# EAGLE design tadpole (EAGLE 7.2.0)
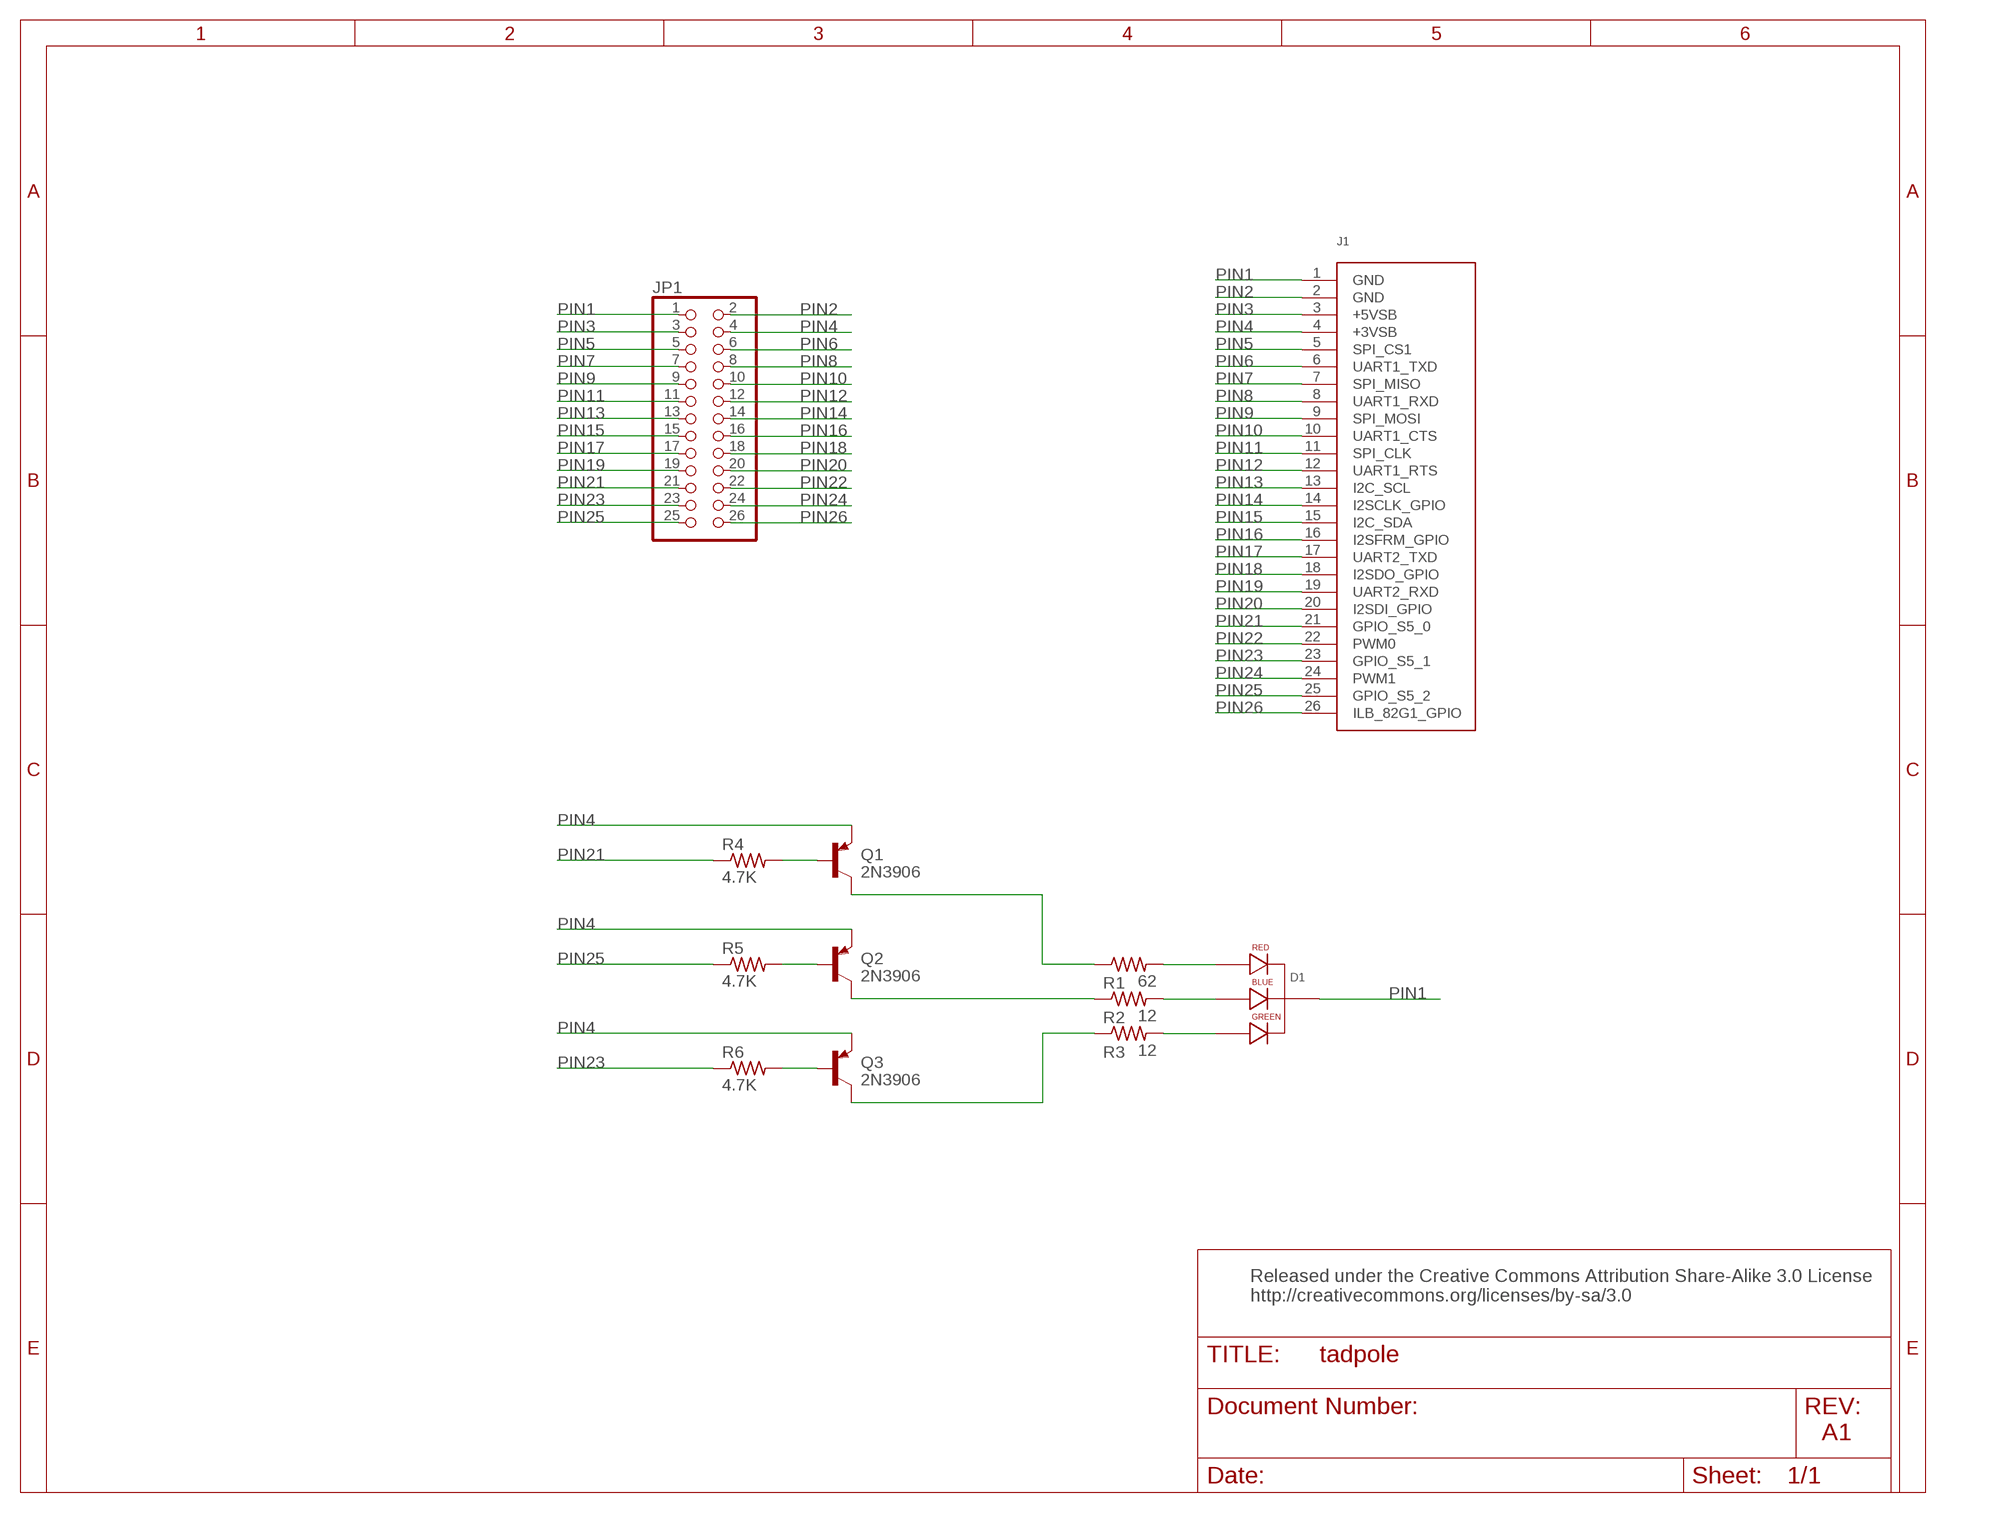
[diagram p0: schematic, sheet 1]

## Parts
D1  LED-RGB-CC-THRUCLEAR  [LED-RGB-THRU]
J1  MBM_LSE  [MBM_LSE]
JP1  PINHD-2X13  [2X13]
Q1  2N3906  [TO92]
Q2  2N3906  [TO92]
Q3  2N3906  [TO92]
R1  62  R-US_0204/5  [0204/5]
R2  12  R-US_0204/5  [0204/5]
R3  12  R-US_0204/5  [0204/5]
R4  4.7K  R-US_0204/5  [0204/5]
R5  4.7K  R-US_0204/5  [0204/5]
R6  4.7K  R-US_0204/5  [0204/5]

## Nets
N$1: Q1.1(C) R1.1
N$2: Q2.1(C) R2.1
N$3: Q3.1(C) R3.1
N$4: Q1.2(B) R4.2
N$5: Q2.2(B) R5.2
N$6: Q3.2(B) R6.2
N$105: D1.1(RED_CATHODE) R1.2
N$106: D1.3(GREEN_CATHODE) R2.2
N$107: D1.4(BLUE_CATHODE) R3.2
PIN1: D1.2(CATHODE) J1.1(GND) JP1.1
PIN2: J1.2(GND) JP1.2
PIN3: J1.3(+5VSB) JP1.3
PIN4: J1.4(+3VSB) JP1.4 Q1.3(E) Q2.3(E) Q3.3(E)
PIN5: J1.5(SPI_CS1) JP1.5
PIN6: J1.6(UART1_TXD) JP1.6
PIN7: J1.7(SPI_MISO) JP1.7
PIN8: J1.8(UART1_RXD) JP1.8
PIN9: J1.9(SPI_MOSI) JP1.9
PIN10: J1.10(UART1_CTS) JP1.10
PIN11: J1.11(SPI_CLK) JP1.11
PIN12: J1.12(UART1_RTS) JP1.12
PIN13: J1.13(I2C_SCL) JP1.13
PIN14: J1.14(I2SCLK_GPIO) JP1.14
PIN15: J1.15(I2C_SDA) JP1.15
PIN16: J1.16(I2SFRM_GPIO) JP1.16
PIN17: J1.17(UART2_TXD) JP1.17
PIN18: J1.18(I2SDO_GPIO) JP1.18
PIN19: J1.19(UART2_RXD) JP1.19
PIN20: J1.20(I2SDI_GPIO) JP1.20
PIN21: J1.21(GPIO_S5_0) JP1.21 R4.1
PIN22: J1.22(PWM0) JP1.22
PIN23: J1.23(GPIO_S5_1) JP1.23 R6.1
PIN24: J1.24(PWM1) JP1.24
PIN25: J1.25(GPIO_S5_2) JP1.25 R5.1
PIN26: J1.26(ILB_82G1_GPIO) JP1.26

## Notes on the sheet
- Released under the Creative Commons Attribution Share-Alike 3.0 License
  http://creativecommons.org/licenses/by-sa/3.0
- A1

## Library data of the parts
D1 = SparkFun-LED:LED-RGB-CC-THRU: RGB Through-hole common cathode LED SparkFun Storefront: COM-00105 (Clear) COM-09264 (Diffuse); PROD_ID: DIO-08418
J1 = mini-lse-lure:MBM_LSE
JP1 = pinhead:PINHD-2X13: PIN HEADER
Q1-Q3 = transistor-pnp:2N3906: PNP Transistor
R1-R6 = resistor:R-US_: RESISTOR, American symbol

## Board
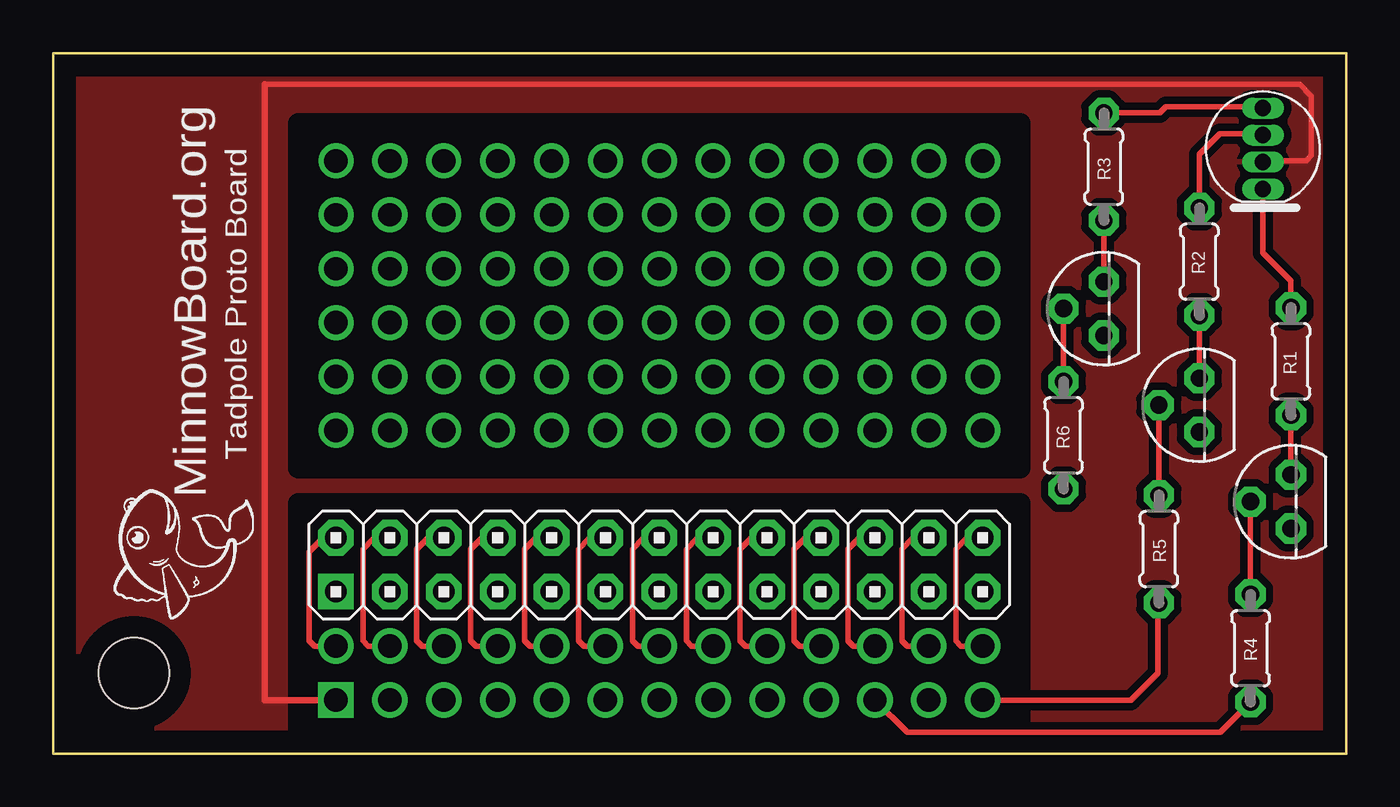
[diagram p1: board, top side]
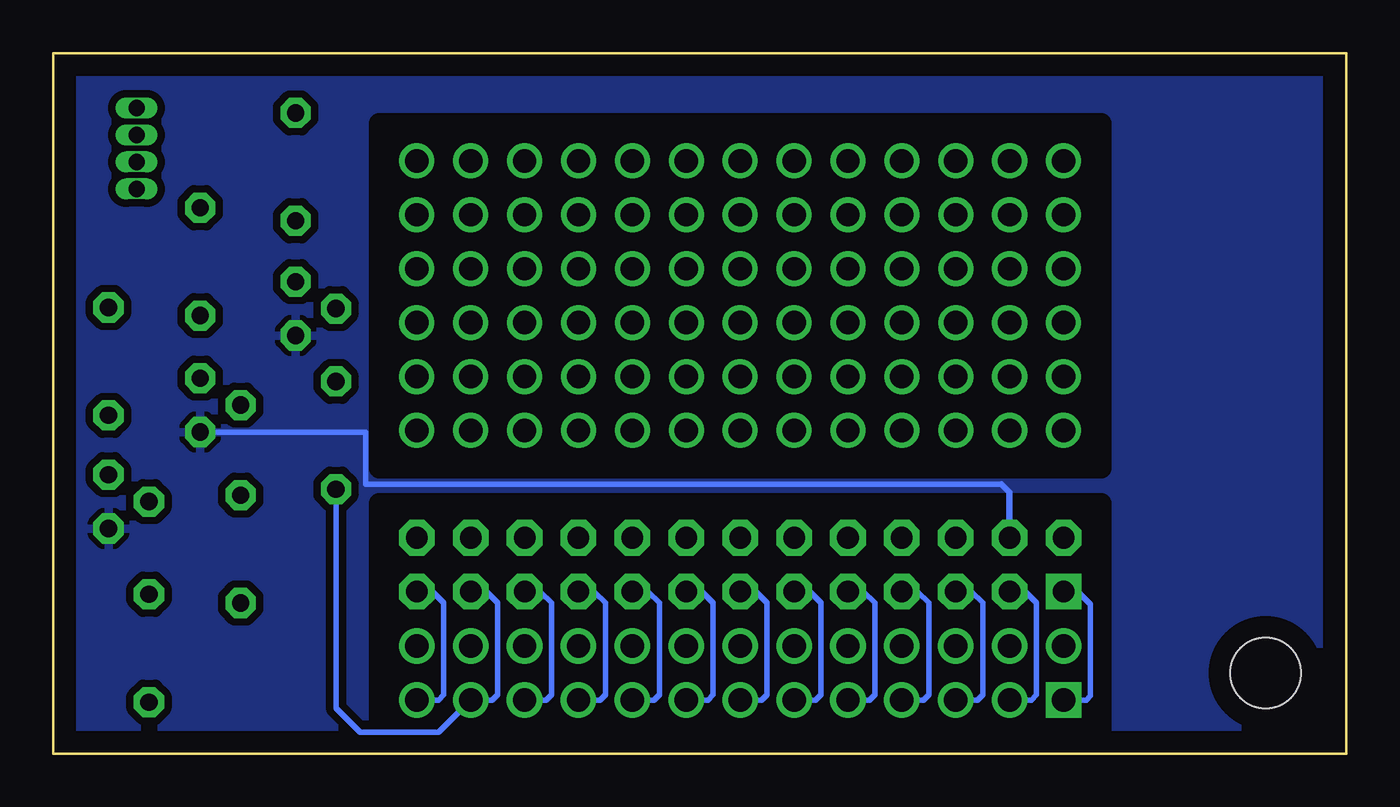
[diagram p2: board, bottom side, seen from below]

Size 60.96 x 33.02 mm. Coordinates in mm from the lower left corner, seen from the top.
Copper layers (1*16): Top 0.035mm / dielectric 1.5mm / Bottom 0.035mm
Design rules "default *": minimum track width 10mil, minimum drill 24mil, track to track 10mil, track to pad 10mil, pad to pad 10mil, via to via 10mil, smd to smd 8mil, copper to edge 40mil, drill to drill 8mil, minimum pad ring 0mil, minimum via ring 8mil, stop-mask expansion 4mil, vias tented up to drill 0mil, thermal gap 10mil
tRestrict: area 11.6,13.5 to 45.6,29.7; area 11.6,0.2 to 45.6,11.8
bRestrict: area 11.6,13.5 to 45.6,29.7; area 11.6,0.3 to 45.6,11.8

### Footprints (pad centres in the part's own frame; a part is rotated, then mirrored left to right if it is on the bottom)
LED-RGB-THRU = drill 0.762 pad 0.889 long: 1 1.905,0; 2 0.635,0; 3 -0.635,0; 4 -1.905,0
MBM_LSE = drill 1.1 pad 1.676 square: 1 -15.24,0 | drill 1.1 pad 1.676: 2 -15.24,2.54; 3 -12.7,0; 4 -12.7,2.54; 5 -10.16,0; 6 -10.16,2.54; 7 -7.62,0; 8 -7.62,2.54; 9 -5.08,0; 10 -5.08,2.54; 11 -2.54,0; 12 -2.54,2.54; 13 0,0; 14 0,2.54; 15 2.54,0; 16 2.54,2.54; 17 5.08,0; 18 5.08,2.54; 19 7.62,0; 20 7.62,2.54; 21 10.16,0; 22 10.16,2.54; 23 12.7,0; 24 12.7,2.54; 25 15.24,0; 26 15.24,2.54 | hole 3.302: -24.765,1.27
2X13 = drill 1.016 pad 1.676 square: 1 -15.24,-1.27 | drill 1.016 pad 1.676 octagon: 2 -15.24,1.27; 3 -12.7,-1.27; 4 -12.7,1.27; 5 -10.16,-1.27; 6 -10.16,1.27; 7 -7.62,-1.27; 8 -7.62,1.27; 9 -5.08,-1.27; 10 -5.08,1.27; 11 -2.54,-1.27; 12 -2.54,1.27; 13 0,-1.27; 14 0,1.27; 15 2.54,-1.27; 16 2.54,1.27; 17 5.08,-1.27; 18 5.08,1.27; 19 7.62,-1.27; 20 7.62,1.27; 21 10.16,-1.27; 22 10.16,1.27; 23 12.7,-1.27; 24 12.7,1.27; 25 15.24,-1.27; 26 15.24,1.27
TO92 = drill 0.813 pad 1.422 octagon: 1 1.27,0; 2 0,1.905; 3 -1.27,0
0204/5 = drill 0.813 pad 1.422 octagon: 1 -2.54,0; 2 2.54,0

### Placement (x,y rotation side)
D1  57.02,28.52 270 top
J1  28.57,2.54 0 top
JP1  28.57,8.92 0 top
Q1  58.34,11.89 90 top
Q2  54.03,16.43 90 top
Q3  49.53,20.98 90 top
R1  58.34,18.49 90 top
R2  54.03,23.19 90 top
R3  49.53,27.66 90 top
R4  56.44,4.98 90 top
R5  52.12,9.65 90 top
R6  47.62,15.01 90 top
U$1  [MINNOWBOARD_LOGO]  9.45,6.05 90 top

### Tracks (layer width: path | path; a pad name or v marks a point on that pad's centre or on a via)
N$1
  Top 0.254: Q1.1 R1.1
N$2
  Top 0.254: Q2.1 R2.1
N$3
  Top 0.254: Q3.1 R3.1
N$4
  Top 0.254: R4.2 Q1.2
N$5
  Top 0.254: R5.2 Q2.2
N$6
  Top 0.254: R6.2 Q3.2
N$14  (via drill 1.1)
  other vias: 13.33,27.94
N$15  (via drill 1.1)
  other vias: 15.87,27.94
N$16  (via drill 1.1)
  other vias: 13.33,15.24
N$17  (via drill 1.1)
  other vias: 15.87,15.24
N$18  (via drill 1.1)
  other vias: 18.41,15.24
N$19  (via drill 1.1)
  other vias: 20.95,15.24
N$20  (via drill 1.1)
  other vias: 23.49,15.24
N$21  (via drill 1.1)
  other vias: 26.03,15.24
N$22  (via drill 1.1)
  other vias: 28.57,15.24
N$23  (via drill 1.1)
  other vias: 31.11,15.24
N$24  (via drill 1.1)
  other vias: 33.65,15.24
N$25  (via drill 1.1)
  other vias: 36.2,15.24
N$26  (via drill 1.1)
  other vias: 38.73,15.24
N$27  (via drill 1.1)
  other vias: 41.27,15.24
N$28  (via drill 1.1)
  other vias: 43.81,15.24
N$29  (via drill 1.1)
  other vias: 18.41,27.94
N$30  (via drill 1.1)
  other vias: 20.95,27.94
N$31  (via drill 1.1)
  other vias: 13.33,17.78
N$32  (via drill 1.1)
  other vias: 15.87,17.78
N$33  (via drill 1.1)
  other vias: 18.41,17.78
N$34  (via drill 1.1)
  other vias: 20.95,17.78
N$35  (via drill 1.1)
  other vias: 23.49,17.78
N$36  (via drill 1.1)
  other vias: 26.03,17.78
N$37  (via drill 1.1)
  other vias: 28.57,17.78
N$38  (via drill 1.1)
  other vias: 31.11,17.78
N$39  (via drill 1.1)
  other vias: 33.65,17.78
N$40  (via drill 1.1)
  other vias: 36.2,17.78
N$41  (via drill 1.1)
  other vias: 38.73,17.78
N$42  (via drill 1.1)
  other vias: 41.27,17.78
N$43  (via drill 1.1)
  other vias: 43.81,17.78
N$44  (via drill 1.1)
  other vias: 23.49,27.94
N$45  (via drill 1.1)
  other vias: 26.03,27.94
N$46  (via drill 1.1)
  other vias: 13.33,20.32
N$47  (via drill 1.1)
  other vias: 15.87,20.32
N$48  (via drill 1.1)
  other vias: 18.41,20.32
N$49  (via drill 1.1)
  other vias: 20.95,20.32
N$50  (via drill 1.1)
  other vias: 23.49,20.32
N$51  (via drill 1.1)
  other vias: 26.03,20.32
N$52  (via drill 1.1)
  other vias: 28.57,20.32
N$53  (via drill 1.1)
  other vias: 31.11,20.32
N$54  (via drill 1.1)
  other vias: 33.65,20.32
N$55  (via drill 1.1)
  other vias: 36.2,20.32
N$56  (via drill 1.1)
  other vias: 38.73,20.32
N$57  (via drill 1.1)
  other vias: 41.27,20.32
N$58  (via drill 1.1)
  other vias: 43.81,20.32
N$59  (via drill 1.1)
  other vias: 28.57,27.94
N$60  (via drill 1.1)
  other vias: 31.11,27.94
N$61  (via drill 1.1)
  other vias: 13.33,22.86
N$62  (via drill 1.1)
  other vias: 15.87,22.86
N$63  (via drill 1.1)
  other vias: 18.41,22.86
N$64  (via drill 1.1)
  other vias: 20.95,22.86
N$65  (via drill 1.1)
  other vias: 23.49,22.86
N$66  (via drill 1.1)
  other vias: 26.03,22.86
N$67  (via drill 1.1)
  other vias: 28.57,22.86
N$68  (via drill 1.1)
  other vias: 31.11,22.86
N$69  (via drill 1.1)
  other vias: 33.65,22.86
N$70  (via drill 1.1)
  other vias: 36.2,22.86
N$71  (via drill 1.1)
  other vias: 38.73,22.86
N$72  (via drill 1.1)
  other vias: 41.27,22.86
N$73  (via drill 1.1)
  other vias: 43.81,22.86
N$74  (via drill 1.1)
  other vias: 33.65,27.94
N$75  (via drill 1.1)
  other vias: 36.2,27.94
N$76  (via drill 1.1)
  other vias: 13.33,25.4
N$77  (via drill 1.1)
  other vias: 15.87,25.4
N$78  (via drill 1.1)
  other vias: 18.41,25.4
N$79  (via drill 1.1)
  other vias: 20.95,25.4
N$80  (via drill 1.1)
  other vias: 23.49,25.4
N$81  (via drill 1.1)
  other vias: 26.03,25.4
N$82  (via drill 1.1)
  other vias: 28.57,25.4
N$83  (via drill 1.1)
  other vias: 31.11,25.4
N$84  (via drill 1.1)
  other vias: 33.65,25.4
N$85  (via drill 1.1)
  other vias: 36.2,25.4
N$86  (via drill 1.1)
  other vias: 38.73,25.4
N$87  (via drill 1.1)
  other vias: 41.27,25.4
N$88  (via drill 1.1)
  other vias: 43.81,25.4
N$89  (via drill 1.1)
  other vias: 38.73,27.94
N$90  (via drill 1.1)
  other vias: 41.27,27.94
N$91  (via drill 1.1)
  other vias: 43.81,27.94
N$105
  Top 0.254: R1.2 58.34,22.3 57.02,23.62 D1.1
N$106
  Top 0.254: R2.2 54.03,28.25 54.99,29.21 56.97,29.21 D1.3
N$107
  Top 0.254: R3.2 52.17,30.2 52.45,30.48 56.97,30.48 D1.4
PIN1
  Top 0.254: 9.98,31.55 58.75,31.55 59.31,30.99 59.31,28.19 59.05,27.94 57.07,27.94 D1.2
  Top 0.305: 9.98,31.55 9.98,2.54 J1.1
  Bottom 0.254: J1.1 12.27,2.54 12.06,2.74 12.06,7.06 12.65,7.64 JP1.1
  pour Top (isolate 0.356): 0,33.02 61.11,33.02 61.11,0 0,0
PIN2
  Top 0.254: J1.2 12.32,5.08 12.06,5.33 12.06,9.53 12.7,10.16 13.31,10.16 JP1.2
PIN3
  Bottom 0.254: J1.3 14.86,2.54 14.6,2.79 14.6,7.11 15.11,7.62 15.85,7.62 JP1.3
PIN4
  Top 0.254: J1.4 14.86,5.08 14.6,5.33 14.6,9.65 15.11,10.16 15.85,10.16 JP1.4
  Bottom 0.254: 16.26,12.7 46.23,12.7 46.23,15.16 Q2.3
  Bottom 0.305: JP1.4 15.87,12.32 16.26,12.7
  pour Bottom (isolate 0.356): 0,33.02 61.01,33.1 61.01,0.08 0,0
PIN5
  Bottom 0.254: J1.5 17.4,2.54 17.14,2.79 17.14,7.11 17.65,7.62 18.39,7.62 JP1.5
PIN6
  Top 0.254: J1.6 17.4,5.08 17.14,5.33 17.14,9.65 17.65,10.16 18.39,10.16 JP1.6
PIN7
  Bottom 0.254: J1.7 19.94,2.54 19.68,2.79 19.68,7.11 20.19,7.62 20.93,7.62 JP1.7
PIN8
  Top 0.254: J1.8 19.94,5.08 19.68,5.33 19.68,9.65 20.19,10.16 20.93,10.16 JP1.8
PIN9
  Bottom 0.254: J1.9 22.48,2.54 22.22,2.79 22.22,7.11 22.73,7.62 23.47,7.62 JP1.9
PIN10
  Top 0.254: J1.10 22.48,5.08 22.22,5.33 22.22,9.65 22.73,10.16 23.47,10.16 JP1.10
PIN11
  Bottom 0.254: J1.11 25.02,2.54 24.76,2.79 24.76,7.11 25.27,7.62 26.01,7.62 JP1.11
PIN12
  Top 0.254: J1.12 25.02,5.08 24.76,5.33 24.76,9.65 25.27,10.16 26.01,10.16 JP1.12
PIN13
  Bottom 0.254: J1.13 27.56,2.54 27.3,2.79 27.3,7.11 27.81,7.62 28.55,7.62 JP1.13
PIN14
  Top 0.254: J1.14 27.56,5.08 27.3,5.33 27.3,9.65 27.81,10.16 28.55,10.16 JP1.14
PIN15
  Bottom 0.254: J1.15 30.1,2.54 29.84,2.79 29.84,7.11 30.35,7.62 31.09,7.62 JP1.15
PIN16
  Top 0.254: J1.16 30.1,5.08 29.84,5.33 29.84,9.65 30.35,10.16 31.09,10.16 JP1.16
PIN17
  Bottom 0.254: J1.17 32.64,2.54 32.38,2.79 32.38,7.11 32.89,7.62 33.63,7.62 JP1.17
PIN18
  Top 0.254: J1.18 32.64,5.08 32.38,5.33 32.38,9.65 32.89,10.16 33.63,10.16 JP1.18
PIN19
  Bottom 0.254: J1.19 35.18,2.54 34.92,2.79 34.92,7.11 35.43,7.62 36.17,7.62 JP1.19
PIN20
  Top 0.254: J1.20 35.18,5.08 34.92,5.33 34.92,9.65 35.43,10.16 36.17,10.16 JP1.20
PIN21
  Top 0.254: J1.21 40.26,1.02 55.02,1.02 R4.1
  Bottom 0.254: J1.21 37.72,2.54 37.46,2.79 37.46,7.11 37.97,7.62 38.71,7.62 JP1.21
PIN22
  Top 0.254: J1.22 37.72,5.08 37.46,5.33 37.46,9.65 37.97,10.16 38.71,10.16 JP1.22
PIN23
  Bottom 0.254: JP1.23 41.25,7.62 40.51,7.62 40,7.11 40,2.79 40.26,2.54 J1.23 42.8,1.02 46.48,1.02 47.62,2.16 R6.1
PIN24
  Top 0.254: J1.24 40.26,5.08 40,5.33 40,9.65 40.51,10.16 41.25,10.16 JP1.24
PIN25
  Top 0.254: J1.25 50.8,2.54 52.07,3.81 52.07,7.06 R5.1
  Bottom 0.254: J1.25 42.8,2.54 42.54,2.79 42.54,7.11 43.05,7.62 43.79,7.62 JP1.25
PIN26
  Top 0.254: J1.26 42.8,5.08 42.54,5.33 42.54,9.65 43.05,10.16 43.79,10.16 JP1.26

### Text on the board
tPlace: R3 | R2 | R1 | Tadpole Proto Board | R6 | MinnowBoard.org | R5 | R4
Notes: Released under the Creative Commons Attribution Share-Alike 3.0 License / http://creativecommons.org/licenses/by-sa/3.0

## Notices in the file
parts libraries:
SparkFun-LED: Licensing: Creative Commons ShareAlike 4.0 International - https://creativecommons.org/licenses/by-sa/4.0
